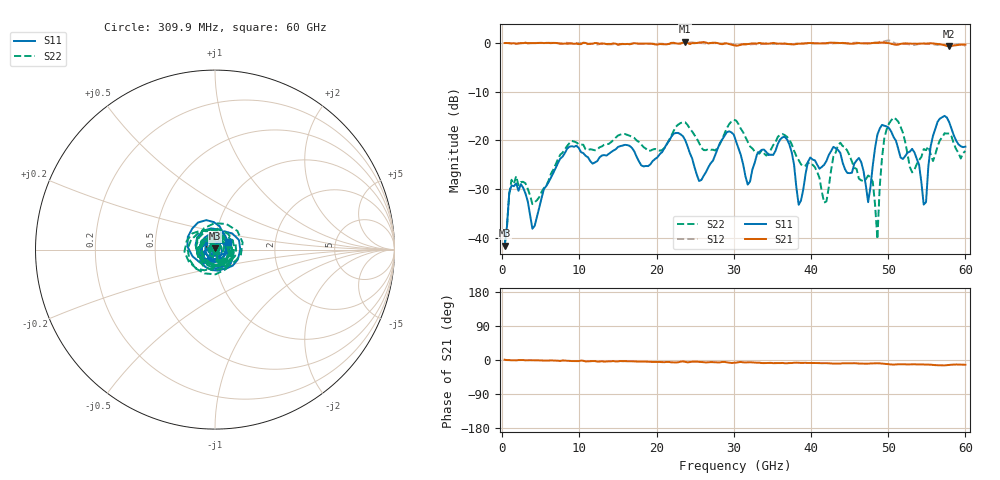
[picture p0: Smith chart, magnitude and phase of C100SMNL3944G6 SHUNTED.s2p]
! 12/11/2024 5:11:06 AM
! D:\C100SMNL3944G6 SHUNTED.S2P
! CHANNEL.1
! TR.MEASUREMENT
! CORRECTED.DATA
# GHZ S RI R 50.0
! FREQ.GHZ  S11RE  S11IM  S21RE  S21IM  S12RE  S12IM  S22RE  S22IM
!; PortSelection: Port_12
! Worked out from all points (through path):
!   200 points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, 309.9 MHz to 60 GHz, reference 50 ohm
!   highest |S21| = 0.30 dB at 23.71 GHz (marker M1); lowest = -0.7 dB at 57.9 GHz (marker M2)
!   group delay of S21, straight-line fit = 575 fs
!   lowest |S11| = -41.7 dB at 309.9 MHz (marker M3), VSWR 1.02, Z = 50.1 + j0.812 ohm
!   |S11| at or under -10 dB: start of sweep to end of sweep
!   |S22| runs from -41.8 to -15.4 dB; largest |S21 - S12| = 0.071
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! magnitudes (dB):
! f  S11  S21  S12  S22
! 309.9 MHz  -41.7  0.0  0.0  -41.8
! 1.21 GHz  -29.3  -0.1  -0.2  -28.1
! 3.909 GHz  -38.2  0.0  0.0  -33.1
! 10.51 GHz  -22.6  0.1  -0.1  -20.9
! 20.41 GHz  -22.9  -0.2  -0.2  -22.1
! 23.71 GHz  -20.0  0.3  0.0  -16.3
! 25.51 GHz  -28.4  0.1  0.0  -20.6
! 30.3 GHz  -20.3  -0.6  -0.4  -16.0
! 31.8 GHz  -29.1  -0.2  -0.3  -20.3
! 36.6 GHz  -19.3  -0.1  -0.2  -18.9
! 38.4 GHz  -33.3  -0.1  -0.1  -24.1
! 40.2 GHz  -24.0  0.0  -0.1  -25.0
! 41.7 GHz  -25.0  -0.1  0.0  -32.8
! 46.2 GHz  -23.6  0.0  0.0  -27.9
! 47.4 GHz  -32.7  -0.1  -0.1  -27.2
! 48.6 GHz  -18.8  0.0  0.1  -40.3
! 49.2 GHz  -16.8  0.1  0.2  -23.6
! 50.1 GHz  -17.5  0.0  0.5  -16.6
! 54.6 GHz  -33.2  -0.1  -0.1  -21.8
! 55.8 GHz  -19.1  -0.1  -0.2  -24.3
! 57.9 GHz  -16.3  -0.7  -0.6  -18.6
! 60 GHz  -21.3  -0.3  -0.6  -22.2
